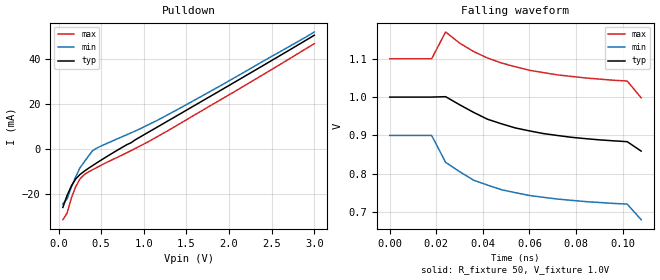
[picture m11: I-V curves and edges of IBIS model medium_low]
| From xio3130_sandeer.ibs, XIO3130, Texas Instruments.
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|[Rising Waveform]
|R_fixture = 50
|V_fixture = 1.0V
|V_fixture_min = 0.9V
|V_fixture_max = 1.1V
|0   0.86200V   0.68000V   1.00000V
|5E-12   0.84760V   0.68180V   1.00700V
|1E-11   0.90810V   0.74120V   1.06700V
|1.5E-11   0.95430V   0.78620V   1.11400V
|2E-11   0.99200V   0.82650V   1.15500V
|2.5E-11   1.02400V   0.85500V   1.18600V
|3E-11   1.05000V   0.88250V   1.21300V
|3.5E-11   1.07200V   0.90210V   1.23400V
|4E-11   1.09000V   0.92120V   1.25300V
|4.5E-11   1.10500V   0.93510V   1.26700V
|5E-11   1.11800V   0.94860V   1.28000V
|5.5E-11   1.12800V   0.95870V   1.29000V
|6E-11   1.13700V   0.96850V   1.29800V
|6.5E-11   1.14500V   0.97590V   1.30500V
|7E-11   1.15100V   0.98310V   1.31200V
|7.5E-11   1.15600V   0.98870V   1.31700V
|8E-11   1.16100V   0.99410V   1.32100V
|8.5E-11   1.16500V   0.99820V   1.32400V
|9E-11   1.16800V   1.00200V   1.32800V
|9.5E-11   1.17100V   1.00500V   1.33000V
|1E-10   1.17300V   1.00800V   1.33200V
|1.05E-10   1.17500V   1.01100V   1.33400V
|1.1E-10   1.17700V   1.01300V   1.33600V
|1.15E-10   1.17900V   1.01500V   1.33700V
|1.2E-10   1.18000V   1.01700V   1.33800V
|1.25E-10   1.18100V   1.01800V   1.33900V
|1.3E-10   1.18200V   1.01900V   1.34000V
|1.35E-10   1.18300V   1.02000V   1.34100V
|1.4E-10   1.18400V   1.02200V   1.34200V
|1.45E-10   1.18500V   1.02200V   1.34200V
|1.5E-10   1.18500V   1.02300V   1.34300V
|1.55E-10   1.18600V   1.02400V   1.34300V
|1.6E-10   1.18600V   1.02500V   1.34300V
|1.65E-10   1.18600V   1.02500V   1.34400V
|1.7E-10   1.18700V   1.02600V   1.34400V
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[Model] medium_low
Model_type Open_drain
Polarity Non-Inverting
Cref = 2.0pF
Rref = 50
Vref = 1.0V
Vmeas =1.0V
|   typ   min   max
C_comp   1.603pF   1.594pF   1.637pF
[Temperature Range]   25   125   -40
[Voltage Range] 1.50V 1.35V 1.65V
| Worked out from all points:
|   falling waveform, R_fixture 50, V_fixture 1.0V: 20-80 % time 60.4ps typ, 70.5ps min, 51.6ps max; typ from 1 V to 0.859 V
| (Process strength) nominal weak strong
[Pulldown]
50mV      -26.04mA   -24.5mA    -31.5mA
100mV     -20.72mA   -22.23mA   -28.52mA
150mV     -16.47mA   -17.03mA   -21.89mA
200mV     -13.42mA   -12.51mA   -16.92mA
250mV     -11.45mA   -8.51mA    -13.4mA
300mV     -9.992mA   -5.886mA   -11.52mA
400mV     -7.42mA    -777uA     -9.271mA
500mV     -4.993mA   1.279mA    -7.277mA
1V        6.212mA    9.729mA    2.111mA
1.2V      10.59mA    13.49mA    6.301mA
1.9V      25.97mA    28.08mA    21.81mA
3V        50.5mA     51.95mA    46.75mA
[Ramp]
| variable   typ   min   max
dV/dt_r 0.1938V/0.0411567ns  0.19662V/0.0449788ns  0.192V/0.0389468ns
dV/dt_f 0.18726V/0.0374755ns  0.1902V/0.0346605ns  0.1854V/0.0369998ns
R_load = 50
[Falling Waveform]
R_fixture = 50
V_fixture = 1.0V
V_fixture_min = 0.9V
V_fixture_max = 1.1V
0s        1V         900mV      1.1V
18ps      1V         900mV      1.1V
24ps      1.001V     829.7mV    1.17V
30ps      980.1mV    805.4mV    1.141V
36ps      960.2mV    783.2mV    1.119V
48ps      930.3mV    758.2mV    1.089V
60ps      911.8mV    743.2mV    1.07V
72ps      899.8mV    733.9mV    1.058V
102ps     883.6mV    720.7mV    1.042V
108ps     859mV      680mV      998mV
